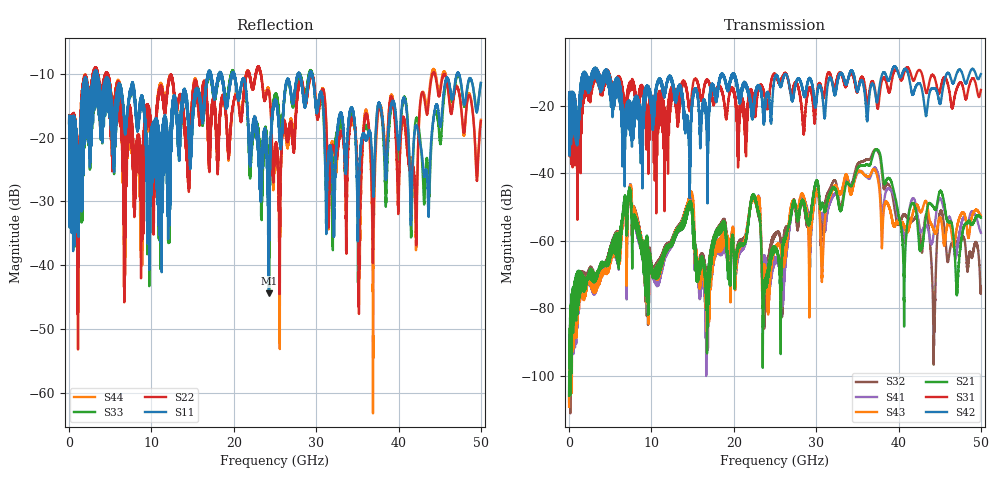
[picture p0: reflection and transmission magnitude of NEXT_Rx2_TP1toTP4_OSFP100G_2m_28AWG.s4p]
! Touchstone data
! Created: 27-Feb-2019 by IdEM 12 (12.1.0)
! COMMENTS
!  Created Wed Feb 27 12:03:36 2019
!  64 Port Network Data from SP1.SP block
!  freq  magS1_1  angS1_1  magS1_2  angS1_2  magS1_3  angS1_3  magS1_4  angS1_4
!  magS1_5  angS1_5  magS1_6  angS1_6  magS1_7  angS1_7  magS1_8  angS1_8
!  magS1_9  angS1_9  magS1_10  angS1_10  magS1_11  angS1_11  magS1_12  angS1_12
!  magS1_13  angS1_13  magS1_14  angS1_14  magS1_15  angS1_15  magS1_16  angS1_16
!  magS1_17  angS1_17  magS1_18  angS1_18  magS1_19  angS1_19  magS1_20  angS1_20
!  magS1_21  angS1_21  magS1_22  angS1_22  magS1_23  angS1_23  magS1_24  angS1_24
!  magS1_25  angS1_25  magS1_26  angS1_26  magS1_27  angS1_27  magS1_28  angS1_28
!  magS1_29  angS1_29  magS1_30  angS1_30  magS1_31  angS1_31  magS1_32  angS1_32
!  magS1_33  angS1_33  magS1_34  angS1_34  magS1_35  angS1_35  magS1_36  angS1_36
!  magS1_37  angS1_37  magS1_38  angS1_38  magS1_39  angS1_39  magS1_40  angS1_40
!  magS1_41  angS1_41  magS1_42  angS1_42  magS1_43  angS1_43  magS1_44  angS1_44
!  magS1_45  angS1_45  magS1_46  angS1_46  magS1_47  angS1_47  magS1_48  angS1_48
!  magS1_49  angS1_49  magS1_50  angS1_50  magS1_51  angS1_51  magS1_52  angS1_52
!  magS1_53  angS1_53  magS1_54  angS1_54  magS1_55  angS1_55  magS1_56  angS1_56
!  magS1_57  angS1_57  magS1_58  angS1_58  magS1_59  angS1_59  magS1_60  angS1_60
!  magS1_61  angS1_61  magS1_62  angS1_62  magS1_63  angS1_63  magS1_64  angS1_64
!  magS2_1  angS2_1  magS2_2  angS2_2  magS2_3  angS2_3  magS2_4  angS2_4
!  magS2_5  angS2_5  magS2_6  angS2_6  magS2_7  angS2_7  magS2_8  angS2_8
!  magS2_9  angS2_9  magS2_10  angS2_10  magS2_11  angS2_11  magS2_12  angS2_12
!  magS2_13  angS2_13  magS2_14  angS2_14  magS2_15  angS2_15  magS2_16  angS2_16
!  magS2_17  angS2_17  magS2_18  angS2_18  magS2_19  angS2_19  magS2_20  angS2_20
!  magS2_21  angS2_21  magS2_22  angS2_22  magS2_23  angS2_23  magS2_24  angS2_24
!  magS2_25  angS2_25  magS2_26  angS2_26  magS2_27  angS2_27  magS2_28  angS2_28
!  magS2_29  angS2_29  magS2_30  angS2_30  magS2_31  angS2_31  magS2_32  angS2_32
!  magS2_33  angS2_33  magS2_34  angS2_34  magS2_35  angS2_35  magS2_36  angS2_36
!  magS2_37  angS2_37  magS2_38  angS2_38  magS2_39  angS2_39  magS2_40  angS2_40
!  magS2_41  angS2_41  magS2_42  angS2_42  magS2_43  angS2_43  magS2_44  angS2_44
!  magS2_45  angS2_45  magS2_46  angS2_46  magS2_47  angS2_47  magS2_48  angS2_48
!  magS2_49  angS2_49  magS2_50  angS2_50  magS2_51  angS2_51  magS2_52  angS2_52
!  magS2_53  angS2_53  magS2_54  angS2_54  magS2_55  angS2_55  magS2_56  angS2_56
!  magS2_57  angS2_57  magS2_58  angS2_58  magS2_59  angS2_59  magS2_60  angS2_60
!  magS2_61  angS2_61  magS2_62  angS2_62  magS2_63  angS2_63  magS2_64  angS2_64
!  magS3_1  angS3_1  magS3_2  angS3_2  magS3_3  angS3_3  magS3_4  angS3_4
!  magS3_5  angS3_5  magS3_6  angS3_6  magS3_7  angS3_7  magS3_8  angS3_8
!  magS3_9  angS3_9  magS3_10  angS3_10  magS3_11  angS3_11  magS3_12  angS3_12
!  magS3_13  angS3_13  magS3_14  angS3_14  magS3_15  angS3_15  magS3_16  angS3_16
!  magS3_17  angS3_17  magS3_18  angS3_18  magS3_19  angS3_19  magS3_20  angS3_20
!  magS3_21  angS3_21  magS3_22  angS3_22  magS3_23  angS3_23  magS3_24  angS3_24
!  magS3_25  angS3_25  magS3_26  angS3_26  magS3_27  angS3_27  magS3_28  angS3_28
!  magS3_29  angS3_29  magS3_30  angS3_30  magS3_31  angS3_31  magS3_32  angS3_32
!  magS3_33  angS3_33  magS3_34  angS3_34  magS3_35  angS3_35  magS3_36  angS3_36
!  magS3_37  angS3_37  magS3_38  angS3_38  magS3_39  angS3_39  magS3_40  angS3_40
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# Hz S MA R 50
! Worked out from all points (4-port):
!   5000 points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, 10 MHz to 50 GHz, reference 50 ohm
!   strongest paths, dB at 10 MHz, 12.51 GHz, 25.01 GHz, 37.51 GHz, 50 GHz:
!     S42: -18.0, -12.5, -11.5, -17.6, -10.7
!     S31: -18.0, -15.9, -10.7, -20.7, -15.4
!     S21: -106.0, -60.9, -62.6, -33.2, -53.2
!     S43: -109.3, -60.4, -62.8, -41.9, -52.7
!     S41: -107.8, -61.3, -65.9, -40.4, -57.7
!     S32: -107.5, -60.1, -58.5, -33.6, -74.3
!   lowest |S11| = -44.4 dB at 24.26 GHz (marker M1), VSWR 1.01, Z = 49.6 - j0.401 ohm
!   |S11| at or under -10 dB: 3.451 GHz to 16.86 GHz (13.4 GHz wide, 132 % of centre); 20.09 GHz to 27.79 GHz (7.695 GHz wide, 32.1 % of centre); 29.5 GHz to 47.1 GHz (17.61 GHz wide, 46 % of centre)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
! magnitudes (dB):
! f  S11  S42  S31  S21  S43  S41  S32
! 10 MHz  -17.7  -18.0  -18.0  -106.0  -109.3  -107.8  -107.5
! 7.41 GHz  -13.1  -19.4  -14.0  -44.6  -43.9  -43.4  -45.2
! 22.88 GHz  -21.5  -14.1  -16.9  -51.1  -48.1  -47.8  -51.4
! 24.26 GHz  -44.4  -17.6  -18.3  -70.1  -75.9  -72.5  -66.7
! 37.23 GHz  -19.3  -17.4  -16.7  -33.0  -39.5  -38.6  -33.0
! 40.67 GHz  -13.7  -9.4  -10.5  -82.1  -55.5  -59.0  -52.3
! 50 GHz  -11.4  -10.7  -15.4  -53.2  -52.7  -57.7  -74.3
